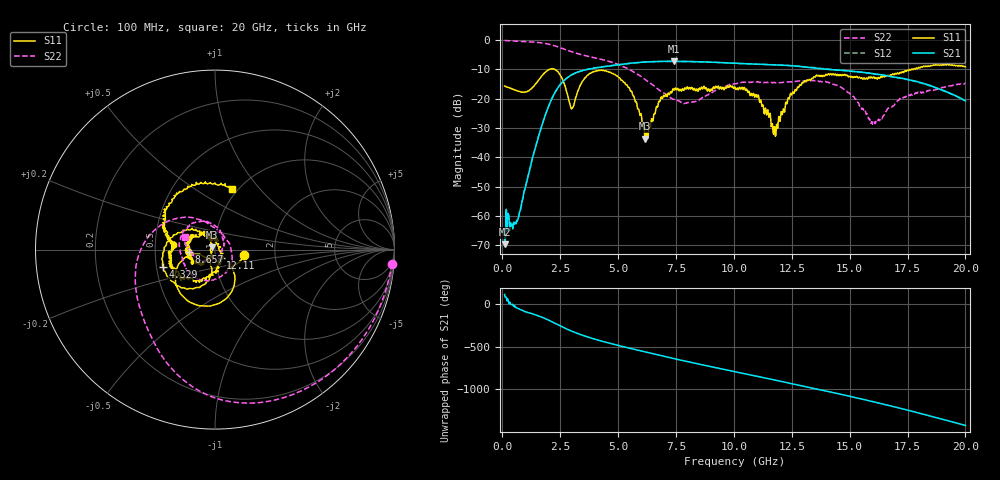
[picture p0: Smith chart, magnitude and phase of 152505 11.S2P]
!  2-Port S-parameters saved by WinCal
! VAR MeasName=S-Parameters (CALIBRATED_DATA) read from VNA (N5230C)
! VAR MeasDate=4/10/2015 9:29:25 AM
! VAR NAME=152505 11
! VAR FILENAME=152505 11.S2P
! VAR DATE=4/10/2015 9:29:25 AM
! VAR PHYS_PORTS=1,2
# Hz S DB R 50
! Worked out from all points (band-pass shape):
!   801 points, 100 MHz to 20 GHz, reference 50 ohm
!   highest |S21| = -7.21 dB at 7.413 GHz (marker M1); lowest = -69.7 dB at 124.9 MHz (marker M2)
!   |S21| within 3 dB of the highest: 3.547 GHz to 14.49 GHz (10.94 GHz wide, 121 % of centre)
!   lowest |S11| = -33.6 dB at 6.17 GHz (marker M3), VSWR 1.04, Z = 48.4 + j1.23 ohm
!   |S11| at or under -10 dB: start of sweep to 2.026 GHz; 2.268 GHz to 17.58 GHz (15.31 GHz wide, 154 % of centre); 17.5963 GHz to 17.66662 GHz (70.32 MHz wide, 0.399 % of centre)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
!   |S22| runs from -28.7 to -0.1 dB; largest |S21 - S12| = 0.0075
!   S11 on the Smith chart (normalised r, x): 100 MHz: 1.39, -0.08; 4.329 GHz: 0.54, -0.11; 8.657 GHz: 0.74, -0.02; 12.11 GHz: 1.06, -0.10; 20 GHz: 0.93, +0.72
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1e8  -15.63 -10.0  -68.15 111.6  -67.16 115.1  -0.08 -4.6
1.24875e8  -15.71 -12.0  -69.73 81.1  -70.33 105.6  -0.11 -5.5
6.72125e8  -17.33 -42.4  -61.11 -52.0  -61.03 -52.3  -0.32 -27.3
2.164625e9  -9.78 -111.6  -19.54 150.2  -19.54 150.4  -1.67 -90.2
2.9855e9  -23.43 -139.3  -11.88 44.1  -11.87 44.2  -3.91 -120.5
3.43325e9  -14.44 -104.9  -10.46 -2.4  -10.43 -2.1  -4.98 -133.9
4.32875e9  -10.34 -161.8  -9.08 -76.7  -9.04 -76.8  -6.64 -162.6
5.497875e9  -16.42 134.3  -7.92 -157.1  -7.90 -157.3  -10.04 151.1
6.1695e9  -33.61 142.6  -7.43 159.2  -7.42 159.0  -13.41 124.0
6.741625e9  -21.38 -133.0  -7.25 122.5  -7.22 122.3  -16.81 103.4
7.41325e9  -17.05 -147.9  -7.21 81.3  -7.20 81.2  -20.17 72.7
8.657e9  -16.67 -174.7  -7.40 8.0  -7.37 7.9  -19.55 -24.4
1.005e10  -15.95 165.3  -7.83 -72.2  -7.88 -72.5  -14.85 -108.1
1.1045e10  -18.69 119.6  -8.19 -127.9  -8.17 -128.0  -14.17 -145.9
1.171662e10  -32.13 31.4  -8.37 -166.4  -8.40 -166.6  -14.49 -163.3
1.211462e10  -24.72 -56.8  -8.55 170.4  -8.52 170.3  -14.39 -172.1
1.338325e10  -13.06 -131.5  -9.42 96.0  -9.32 96.2  -13.80 155.1
1.497525e10  -12.40 179.5  -10.49 2.0  -10.49 2.0  -17.97 84.5
1.599512e10  -12.96 172.6  -11.41 -62.0  -11.44 -62.4  -28.75 -15.7
1.669162e10  -12.21 171.4  -12.23 -107.3  -12.31 -108.6  -23.16 -112.9
1.853238e10  -8.68 130.4  -15.61 125.1  -15.83 124.4  -17.09 -175.6
2e10  -9.08 74.6  -20.70 18.7  -20.71 19.2  -14.83 157.0
